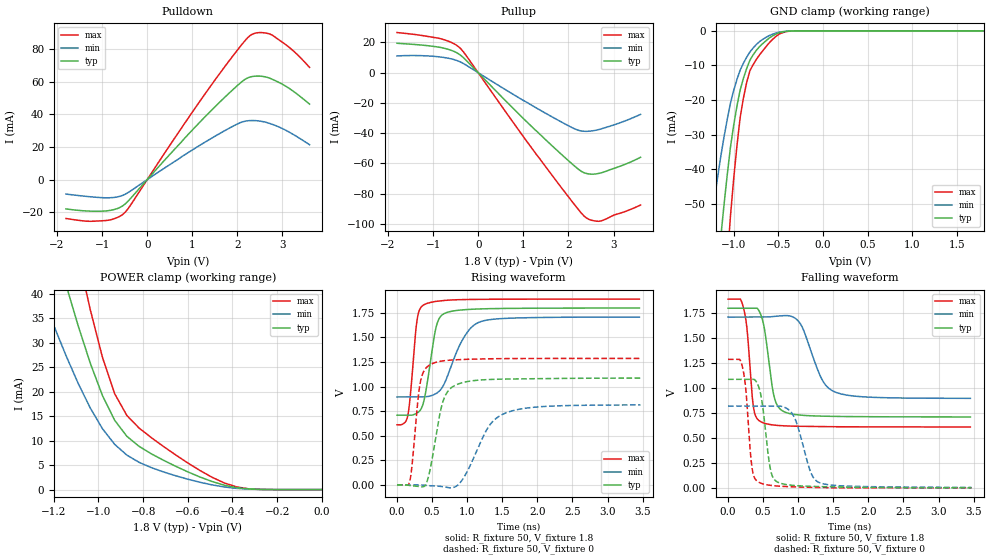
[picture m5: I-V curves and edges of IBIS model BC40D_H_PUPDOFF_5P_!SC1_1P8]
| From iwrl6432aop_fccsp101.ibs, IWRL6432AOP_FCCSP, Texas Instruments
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|   Model Cell BC40D_H_PUPDOFF_5P_!SC1_1P8
|BC40D_H_PUPDOFF_5P_!SC1_1P8
[Model]   BC40D_H_PUPDOFF_5P_!SC1_1P8
Model_type   I/O
Polarity   Non-Inverting
Enable   Active-Low
Vinl =  0.63
Vinh =  1.17
Cref =  15pF
Rref =  100.0000M
Vref =  0V
Vmeas =  0.9
C_comp   2.364487p   2.290698p   2.389419p
|[Input load] weak_pupdoff
|[Output drive] fast
|[supplytol] 5
|[temp] ind
[Model Spec]
Vinl   0.63   0.5985   0.6615
Vinh   1.17   1.1115   1.2285
[Temperature Range]   25   125   -40
[Voltage Range]   1.8   1.71   1.89
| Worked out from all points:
|   slope of the pulldown table from 0 to 0.27 V, typ, clamps not added: 32.2 ohm
|   slope of the pullup table from 0 to 0.27 V, typ, clamps not added: 32.5 ohm
|   GND clamp passes 1 mA (typ) near -0.53 V on its own axis
|   POWER clamp passes 1 mA (typ) near -0.44 V on its own axis
|   rising waveform, R_fixture 50, V_fixture 1.8: 20-80 % time 145ps typ, 303ps min, 93.6ps max; typ from 0.709 V to 1.8 V
|   rising waveform, R_fixture 50, V_fixture 0: 20-80 % time 176ps typ, 352ps min, 106ps max; typ from 0 V to 1.09 V
|   falling waveform, R_fixture 50, V_fixture 1.8: 20-80 % time 130ps typ, 266ps min, 88.3ps max; typ from 1.8 V to 0.71 V
|   falling waveform, R_fixture 50, V_fixture 0: 20-80 % time 113ps typ, 198ps min, 84.5ps max; typ from 1.09 V to 0 V
| Nom Voltages:
|   VDD=1.1, VDDS=1.8, VDDS18=1.8, ESD_BIASFET=0, VSS=0, VSSS=0
| Min Voltages:
|   VDD=1.045, VDDS=1.71, VDDS18=1.71, ESD_BIASFET=0, VSS=0, VSSS=0
| Max Voltages:
|   VDD=1.16, VDDS=1.89, VDDS18=1.89, ESD_BIASFET=0, VSS=0, VSSS=0
[POWER_clamp]
|   voltage   I(typ)   I(min)   I(max)
-1.8V     158.8mA    112.5mA    219.7mA
-1.255V   59.93mA    39.99mA    84.86mA
-1.127V   39.08mA    25.5mA     55.75mA
-1.055V   28.36mA    18.34mA    40.41mA
-981.8mV  19.18mA    12.43mA    26.98mA
-927.3mV  14.16mA    9.239mA    19.58mA
-872.7mV  10.89mA    7.049mA    15.14mA
-818.2mV  8.843mA    5.579mA    12.59mA
-600mV    3.63mA     2.128mA    5.45mA
-436.4mV  903.9uA    539uA      1.358mA
-327.3mV  138.2uA    94.87uA    160.3uA
0V        19.3nA     133.7nA    230.3nA
[Pulldown]
|   voltage   I(typ)   I(min)   I(max)
-1.8V     -17.92mA   -8.85mA    -23.8mA
-1.309V   -19.26mA   -10.37mA   -25.5mA
-927.3mV  -19.22mA   -11.12mA   -25.08mA
-654.5mV  -17.65mA   -10.56mA   -23.13mA
-490.9mV  -14.97mA   -8.985mA   -20.05mA
1.364V    40.78mA    24.32mA    55.7mA
2.073V    59.41mA    35mA       81.91mA
2.291V    62.96mA    36.2mA     88.48mA
2.509V    63.41mA    35.84mA    90.12mA
2.782V    61.38mA    33.82mA    88.42mA
3.218V    54.59mA    28.02mA    79.45mA
3.6V      46.26mA    21.39mA    68.79mA
[Pullup]
|   voltage   I(typ)   I(min)   I(max)
-1.8V     19.47mA    11.11mA    26.55mA
-818.2mV  16.61mA    10.32mA    22.37mA
-545.5mV  14.21mA    8.765mA    19.31mA
-381.8mV  11.35mA    6.928mA    15.71mA
1.255V    -37.58mA   -22.7mA    -52.59mA
2.127V    -61.49mA   -36.97mA   -86.91mA
2.291V    -65.3mA    -38.55mA   -92.97mA
2.4V      -66.65mA   -38.77mA   -96.07mA
2.564V    -67.08mA   -38.3mA    -97.93mA
2.727V    -66.24mA   -37.15mA   -97.99mA
3.273V    -60.4mA    -31.68mA   -91.65mA
3.6V      -55.92mA   -27.55mA   -87.52mA
[GND_clamp]
|   voltage   I(typ)   I(min)   I(max)
-1.8V     -270.2mA   -170.2mA   -430.1mA
-1.255V   -91.66mA   -55.91mA   -148.4mA
-1.145V   -59.91mA   -36.45mA   -97.09mA
-1.109V   -50.48mA   -30.83mA   -81.55mA
-1.073V   -41.73mA   -25.65mA   -67.05mA
-1.036V   -33.66mA   -20.92mA   -53.59mA
-927.3mV  -17.07mA   -11.35mA   -25.04mA
-854.5mV  -10.86mA   -7.617mA   -14.91mA
-781.8mV  -6.919mA   -4.945mA   -9.771mA
-636.4mV  -2.823mA   -1.868mA   -4.529mA
-381.8mV  -84.73uA   -78.82uA   -126.1uA
1.8V      19.3nA     350.9nA    215.8nA
[Ramp]
| variable   typ   min   max
dV/dt_f 0.66537461/0.1328587n 0.49951599/0.27202412n  0.7771902/89.861739p
dV/dt_r  0.6647348/0.17860803n 0.51000261/0.36733301n 0.78144821/0.10715466n
R_load = 50
[Rising Waveform]
R_fixture = 50
V_fixture = 1.8
V_fixture_min = 1.71
V_fixture_max = 1.89
|   time   V(typ)   V(min)   V(max)
0s        709.2mV    894.4mV    611.3mV
151.7ps   709.2mV    894.4mV    699.2mV
187ps     709.2mV    894.4mV    887.5mV
285.9ps   730.7mV    894.4mV    1.677V
389ps     873.4mV    896.1mV    1.835V
553.8ps   1.596V     928.7mV    1.867V
686.1ps   1.748V     1.049V     1.877V
948.8ps   1.782V     1.496V     1.886V
1.197ns   1.791V     1.662V     1.888V
3.453ns   1.8V       1.708V     1.89V
[Rising Waveform]
R_fixture = 50
V_fixture = 0
V_fixture_min = 0
V_fixture_max = 0
|   time   V(typ)   V(min)   V(max)
0s        0V         0V         0V
177.7ps   -5.678mV   0V         25.83mV
328.8ps   -18.26mV   0V         1.031V
407.1ps   0V         -4.568mV   1.184V
481.7ps   192mV      -8.475mV   1.227V
655.2ps   850.1mV    -18.02mV   1.262V
852.1ps   1.021V     -9.072mV   1.273V
1.295ns   1.072V     580.9mV    1.283V
1.529ns   1.077V     726.3mV    1.285V
3.47ns    1.087V     813.6mV    1.287V
[Falling Waveform]
R_fixture = 50
V_fixture = 1.8
V_fixture_min = 1.71
V_fixture_max = 1.89
|   time   V(typ)   V(min)   V(max)
0s        1.799V     1.711V     1.891V
218.1ps   1.799V     1.711V     1.81V
270.7ps   1.799V     1.711V     1.592V
365.8ps   1.799V     1.711V     794.1mV
472.5ps   1.724V     1.711V     660.3mV
652.7ps   925.8mV    1.717V     629.1mV
801.2ps   762mV      1.726V     621.2mV
1.032ns   728.7mV    1.643V     616.6mV
1.52ns    715.8mV    962mV      612.3mV
3.453ns   710.3mV    896.7mV    610mV
[Falling Waveform]
R_fixture = 50
V_fixture = 0
V_fixture_min = 0
V_fixture_max = 0
|   time   V(typ)   V(min)   V(max)
0s        1.087V     819.6mV    1.287V
203.8ps   1.087V     819.6mV    1.216V
254.1ps   1.087V     819.6mV    983.5mV
341.4ps   1.087V     819.6mV    205.8mV
444.1ps   997.6mV    819.6mV    54.23mV
601.9ps   194.9mV    819.6mV    25.35mV
714.7ps   54.87mV    819.6mV    17.53mV
935.6ps   24.13mV    720mV      10.14mV
1.302ns   12.55mV    52.42mV    3.16mV
3.47ns    0V         4.122mV    0V
